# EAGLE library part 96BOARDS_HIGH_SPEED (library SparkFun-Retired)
96 BOARDS high speed connectors. 2 variants: 1. "TOP" goes on the top of the board, called a "Receptacale" in the parlance. Candidate parts would be FCI/Bergquist 61082-061409LF 2. "BOTTOM" goes on the bottom of a board. Candidate parts would be FCI 61083-063409LF for 7mm board-to-board clearance, or 61083-064409LF for 8mm clearance. If you're placing one on the bottom of a board, take care to mind the pin-1 orientation.
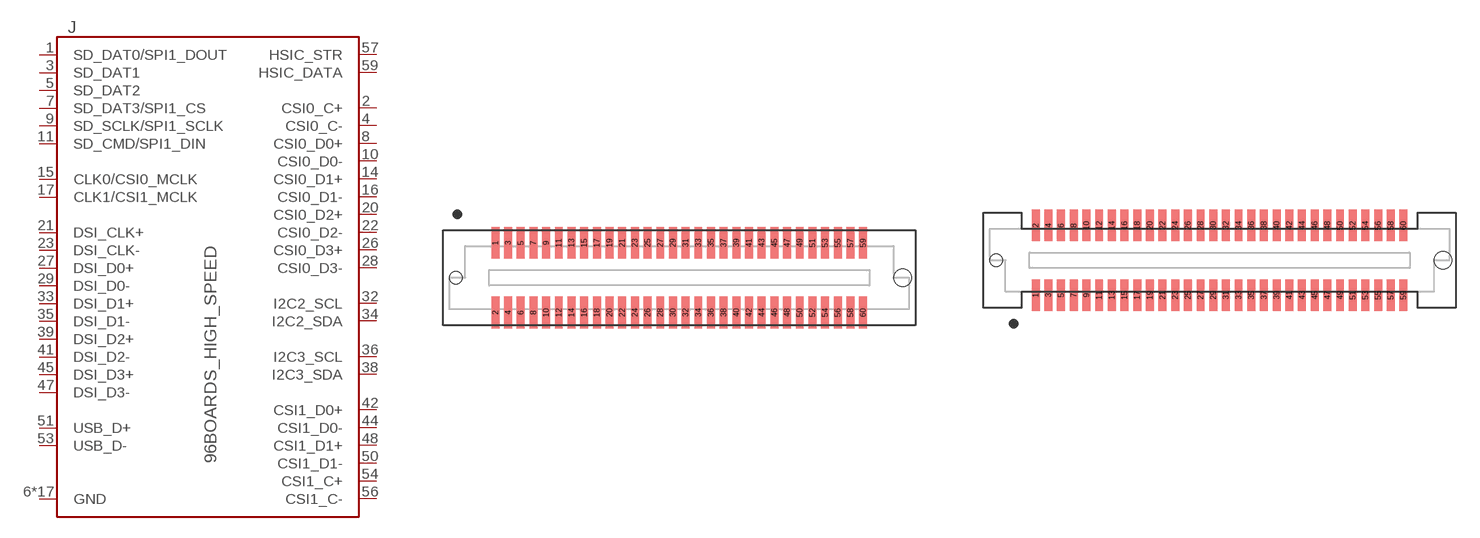
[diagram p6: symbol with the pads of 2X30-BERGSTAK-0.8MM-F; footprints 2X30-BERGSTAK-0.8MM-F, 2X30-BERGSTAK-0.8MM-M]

Designator prefix J

## 96BOARDS_HIGH_SPEEDBOTTOM (VALUE: 96BOARDS HIGH SPEED)  [2X30-BERGSTAK-0.8MM-F]
1  SD_DAT0/SPI1_DOUT
2  CSI0_C+
3  SD_DAT1
4  CSI0_C-
5  SD_DAT2
6  GND
7  SD_DAT3/SPI1_CS
8  CSI0_D0+
9  SD_SCLK/SPI1_SCLK
10  CSI0_D0-
11  SD_CMD/SPI1_DIN
12  GND
13  GND
14  CSI0_D1+
15  CLK0/CSI0_MCLK
16  CSI0_D1-
17  CLK1/CSI1_MCLK
18  GND
19  GND
20  CSI0_D2+
21  DSI_CLK+
22  CSI0_D2-
23  DSI_CLK-
24  GND
25  GND
26  CSI0_D3+
27  DSI_D0+
28  CSI0_D3-
29  DSI_D0-
30  GND
31  GND
32  I2C2_SCL
33  DSI_D1+
34  I2C2_SDA
35  DSI_D1-
36  I2C3_SCL
37  GND
38  I2C3_SDA
39  DSI_D2+
40  GND
41  DSI_D2-
42  CSI1_D0+
43  GND
44  CSI1_D0-
45  DSI_D3+
46  GND
47  DSI_D3-
48  CSI1_D1+
49  GND
50  CSI1_D1-
51  USB_D+
52  GND
53  USB_D-
54  CSI1_C+
55  GND
56  CSI1_C-
57  HSIC_STR
58  GND
59  HSIC_DATA

## 96BOARDS_HIGH_SPEEDTOP (VALUE: 96 BOARDS HIGH SPEED)  [2X30-BERGSTAK-0.8MM-M]
Pads as for 2X30-BERGSTAK-0.8MM-F

## Footprint 2X30-BERGSTAK-0.8MM-F (pad centres in mm)
96BOARDS High Speed connector For video & camera interfaces Part as drawn in the for the part: - FCI 61083-063402PLF for 7mm stack height or - FCI 61083-064402PLF for 8mm stack
smd 0.5 x 2: 1 -11.6,2.2; 2 -11.6,-2.2; 3 -10.8,2.2; 4 -10.8,-2.2; 5 -10,2.2; 6 -10,-2.2; 7 -9.2,2.2; 8 -9.2,-2.2; 9 -8.4,2.2; 10 -8.4,-2.2; 11 -7.6,2.2; 12 -7.6,-2.2; 13 -6.8,2.2; 14 -6.8,-2.2; 15 -6,2.2; 16 -6,-2.2; 17 -5.2,2.2; 18 -5.2,-2.2; 19 -4.4,2.2; 20 -4.4,-2.2; 21 -3.6,2.2; 22 -3.6,-2.2; 23 -2.8,2.2; 24 -2.8,-2.2; 25 -2,2.2; 26 -2,-2.2; 27 -1.2,2.2; 28 -1.2,-2.2; 29 -0.4,2.2; 30 -0.4,-2.2; 31 0.4,2.2; 32 0.4,-2.2; 33 1.2,2.2; 34 1.2,-2.2; 35 2,2.2; 36 2,-2.2; 37 2.8,2.2; 38 2.8,-2.2; 39 3.6,2.2; 40 3.6,-2.2; 41 4.4,2.2; 42 4.4,-2.2; 43 5.2,2.2; 44 5.2,-2.2; 45 6,2.2; 46 6,-2.2; 47 6.8,2.2; 48 6.8,-2.2; 49 7.6,2.2; 50 7.6,-2.2; 51 8.4,2.2; 52 8.4,-2.2; 53 9.2,2.2; 54 9.2,-2.2; 55 10,2.2; 56 10,-2.2; 57 10.8,2.2; 58 10.8,-2.2; 59 11.6,2.2; 60 11.6,-2.2
hole 0.8 at -14.1,0
hole 1.12 at 14.1,0

## Footprint 2X30-BERGSTAK-0.8MM-M (pad centres in mm)
smd 0.5 x 2: 1 -11.6,-2.2; 2 -11.6,2.2; 3 -10.8,-2.2; 4 -10.8,2.2; 5 -10,-2.2; 6 -10,2.2; 7 -9.2,-2.2; 8 -9.2,2.2; 9 -8.4,-2.2; 10 -8.4,2.2; 11 -7.6,-2.2; 12 -7.6,2.2; 13 -6.8,-2.2; 14 -6.8,2.2; 15 -6,-2.2; 16 -6,2.2; 17 -5.2,-2.2; 18 -5.2,2.2; 19 -4.4,-2.2; 20 -4.4,2.2; 21 -3.6,-2.2; 22 -3.6,2.2; 23 -2.8,-2.2; 24 -2.8,2.2; 25 -2,-2.2; 26 -2,2.2; 27 -1.2,-2.2; 28 -1.2,2.2; 29 -0.4,-2.2; 30 -0.4,2.2; 31 0.4,-2.2; 32 0.4,2.2; 33 1.2,-2.2; 34 1.2,2.2; 35 2,-2.2; 36 2,2.2; 37 2.8,-2.2; 38 2.8,2.2; 39 3.6,-2.2; 40 3.6,2.2; 41 4.4,-2.2; 42 4.4,2.2; 43 5.2,-2.2; 44 5.2,2.2; 45 6,-2.2; 46 6,2.2; 47 6.8,-2.2; 48 6.8,2.2; 49 7.6,-2.2; 50 7.6,2.2; 51 8.4,-2.2; 52 8.4,2.2; 53 9.2,-2.2; 54 9.2,2.2; 55 10,-2.2; 56 10,2.2; 57 10.8,-2.2; 58 10.8,2.2; 59 11.6,-2.2; 60 11.6,2.2
hole 0.8 at -14.1,0
hole 1.12 at 14.1,0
